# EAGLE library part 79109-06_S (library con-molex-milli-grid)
RECEPTACAL
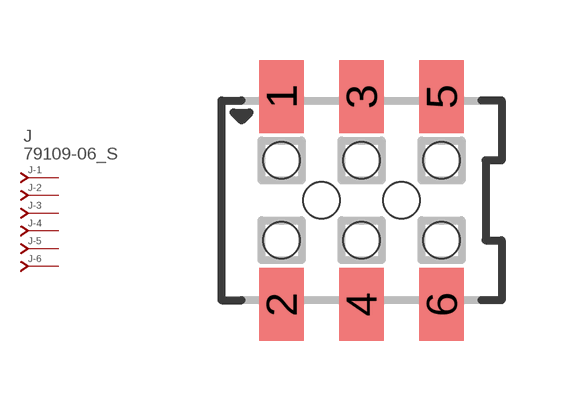
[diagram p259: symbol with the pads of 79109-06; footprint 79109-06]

Designator prefix J; gates -1=J-NV -2=J-N -3=J-N -4=J-N -5=J-N -6=J-N

## 79109-06_S  [79109-06]
1  -1:J  pas
2  -2:J  pas
3  -3:J  pas
4  -4:J  pas
5  -5:J  pas
6  -6:J  pas

## Footprint 79109-06 (pad centres in mm)
RECEPTACAL SMD Dual Row, Vertical, Pass-Thru
smd 1.12 x 1.83: 1 -2,2.6; 2 -2,-2.6; 3 0,2.6; 4 0,-2.6; 5 2,2.6; 6 2,-2.6
hole 0.914 at -1,0
hole 0.914 at -2,1
hole 0.914 at -2,-1
hole 0.914 at 0,-1
hole 0.914 at 0,1
hole 0.914 at 2,-1
hole 0.914 at 2,1
hole 0.914 at 1,0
